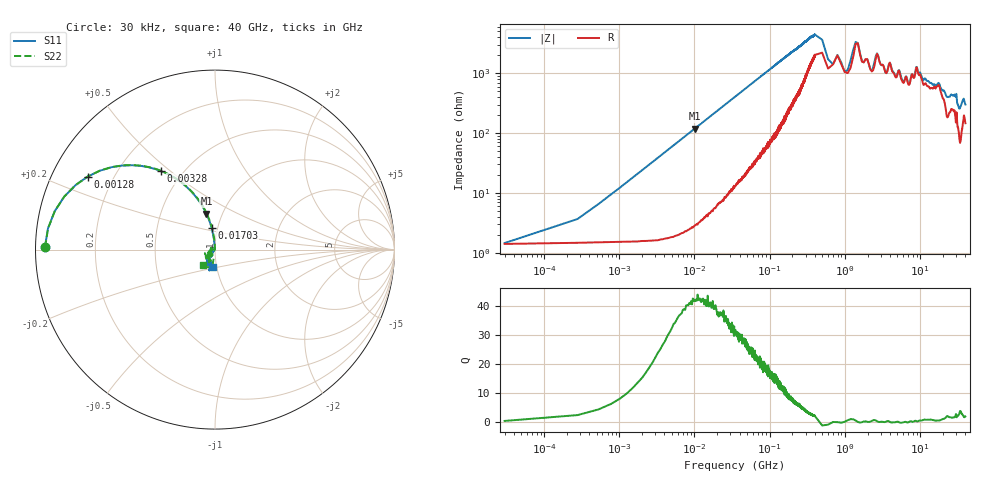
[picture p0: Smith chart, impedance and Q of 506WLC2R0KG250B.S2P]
!  American Technical Ceramics  Date:  9/12/2011
!  One Norden Lane
!  Huntington Station,  NY.  11746-2102
!  Tel:  (631) 622-4700  Fax:  (631) 622-4748
!  Part Number  506WLC2R0KG250B
!  Description:  Ultra-Broadband Inductor
!  Application:  Ultra-broadband DC block decoupling, bias tee
# GHZ S DB R 50
! Freq  |S11|  S11 Ph  |S21|  S21 Ph  |S12|  S12 Ph  |S22|  S22 Ph
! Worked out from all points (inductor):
!   2000 points, 30 kHz to 40 GHz, reference 50 ohm
!   read as one part in shunt: L = 1.89 uH near 2.53 MHz
!   highest Q = 42.2 at 10.03 MHz (marker M1), where L = 1.88 uH
!   self-resonance near 400 MHz
!   S11 on the Smith chart (normalised r, x): 30 kHz: 0.03, +0.01; 1.28 MHz: 0.11, +0.26; 3.28 MHz: 0.38, +0.46; 17.03 MHz: 0.94, +0.23; 40 GHz: 0.96, -0.19
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3e-05  -0.46 179.2  -25.18 14.0  -25.18 14.0  -0.47 179.2
0.00053  -0.74 166.5  -12.41 63.3  -12.40 63.3  -0.74 166.5
0.00128  -1.75 150.2  -6.01 54.4  -6.01 54.4  -1.75 150.1
0.00328  -5.50 124.5  -1.66 32.0  -1.66 32.0  -5.50 124.3
0.00353  -5.94 122.6  -1.47 30.2  -1.47 30.2  -5.95 122.4
0.01003  -13.75 103.4  -0.23 11.8  -0.23 11.8  -13.76 102.8
0.01703  -18.19 98.9  -0.10 7.1  -0.10 7.1  -18.21 97.9
0.03478  -24.35 96.2  -0.04 3.5  -0.04 3.5  -24.37 94.1
0.13852  -37.43 98.8  -0.02 1.0  -0.01 1.0  -37.53 91.9
0.32576  -50.60 163.3  -0.02 0.7  -0.01 0.7  -54.59 151.5
0.3635  -49.37 -169.0  -0.01 0.7  -0.02 0.7  -53.28 -165.0
0.39725  -48.15 -154.8  -0.02 0.7  -0.02 0.7  -50.69 -148.9
0.4  -48.03 -154.0  -0.02 0.7  -0.02 0.7  -50.50 -148.2
3.865  -34.87 -137.4  -0.14 0.8  -0.14 0.8  -32.64 -160.3
7.33  -25.39 -135.4  -0.26 2.6  -0.24 2.6  -25.23 -136.7
13.072  -25.85 -137.8  -0.22 3.7  -0.21 3.7  -31.02 -139.1
17.032  -21.69 -116.0  -0.29 5.6  -0.28 5.6  -23.16 -113.5
23.17  -25.60 -136.3  -0.14 7.6  -0.14 7.6  -28.20 -157.0
29.308  -21.77 -112.3  -0.11 10.1  -0.09 10.1  -22.43 -115.2
34.555  -23.48 -123.8  -0.11 11.8  -0.10 11.8  -31.58 -136.7
37.426  -18.74 -106.0  -0.15 12.7  -0.15 12.7  -21.14 -102.7
40  -20.01 -97.0  -0.20 13.5  -0.21 13.5  -19.24 -127.0
